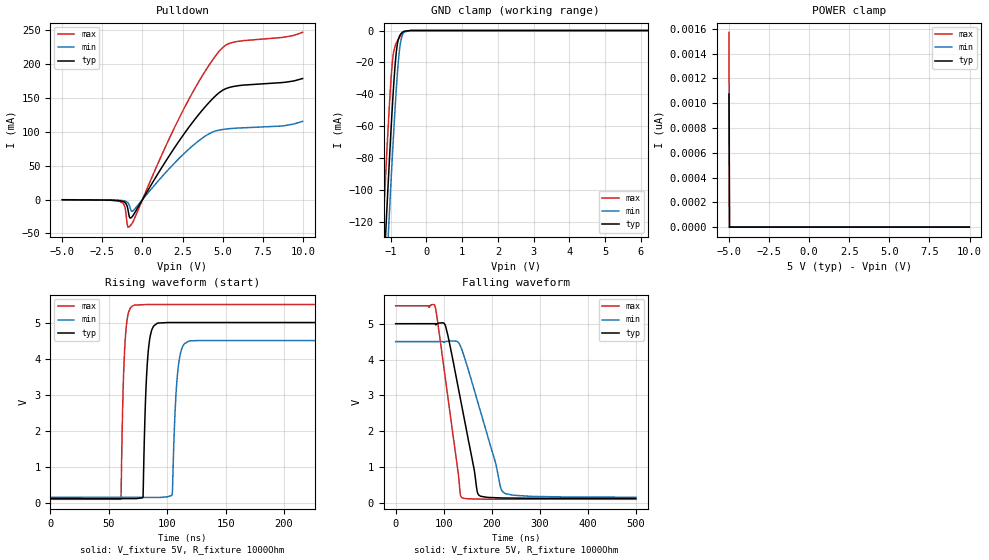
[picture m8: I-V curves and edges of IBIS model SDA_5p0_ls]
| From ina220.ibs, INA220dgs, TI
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|   Model
[Model]   SDA_5p0_ls
Model_type   I/O_open_drain
Polarity   Non-Inverting
Enable   Active-Low
Vinl = 1.5
Vinh = 3.5
Vmeas = 2.5
Vref = 5
Cref = 1pF
Rref = 1000
|   typ   min   max
C_comp   2.1193190E-12   1.8449300E-12 2.3639330E-12
[Voltage Range]   5   4.5   5.5
[Temperature Range]   27   85   -40
[Pullup Reference]   5   4.5   5.5
[Pulldown Reference]   -0   -0   -0
[Power Clamp Reference]   5   4.5   5.5
[GND Clamp Reference]   -0   -0   -0
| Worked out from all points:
|   slope of the pulldown table from 0 to 0.75 V, typ, clamps not added: 25.1 ohm
|   GND clamp passes 1 mA (typ) near -0.67 V on its own axis
|   falling waveform, V_fixture 5V, R_fixture 1000Ohm: 20-80 % time 42.4ns typ, 56.4ns min, 32.8ns max; typ from 5 V to 0.121 V
|   rising waveform, V_fixture 5V, R_fixture 1000Ohm: 20-80 % time 3.38ns typ, 3.94ns min, 2.89ns max; typ from 0.12 V to 5 V
[Pulldown]
|   Voltage   I(typ)   I(min)   I(max)
-5V       -196.2uA   -134.4uA   -251uA
-1.25V    -2.441mA   -1.382mA   -4.492mA
-1.085V   -4.401mA   -2.153mA   -12.11mA
-965mV    -9.014mA   -3.516mA   -34.28mA
-830mV    -24.29mA   -7.959mA   -40.07mA
-710mV    -26.92mA   -16.23mA   -37.21mA
-575mV    -23.01mA   -16.32mA   -31.97mA
2.47V     92.88mA    65.15mA    128.9mA
3.94V     137.8mA    94.18mA    190.8mA
4.78V     157.9mA    102.6mA    219mA
5.62V     166.8mA    105.1mA    232mA
9.985V    178.8mA    115.6mA    247mA
[GND Clamp]
|   Voltage   I(typ)   I(min)   I(max)
-5V       -2.019A    -2.05A     -1.986A
-1.25V    -176mA     -210.3mA   -138.9mA
-1.145V   -127.9mA   -162mA     -91.29mA
-1.1V     -107.8mA   -141.6mA   -71.72mA
-1.055V   -88.14mA   -121.6mA   -53.09mA
-965mV    -51.09mA   -82.91mA   -22.18mA
-920mV    -34.59mA   -64.52mA   -13.48mA
-860mV    -16.84mA   -41.85mA   -8.642mA
-800mV    -6.709mA   -22.67mA   -5.926mA
-740mV    -2.824mA   -9.434mA   -3.68mA
-620mV    -430.2uA   -885.3uA   -725.2uA
9.985V    0A         0A         0A
[POWER Clamp]
|   Voltage   I(typ)   I(min)   I(max)
-5V       1.074nA    0A         1.571nA
-4.97V    0A         0A         0A
-4.955V   0A         0A         0A
9.985V    0A         0A         0A
[Ramp]
R_load = 1000
|   typ   min   max
dV/dt_r   2.92774/3.37213e-09   2.60948/3.92775e-09   3.24271/2.87247e-09
dV/dt_f   2.9275/4.23604e-08   2.60776/5.64045e-08   3.24268/3.27444e-08
[Falling Waveform]
V_fixture = 5V
V_fixture_min = 4.5V
V_fixture_max = 5.5V
R_fixture = 1000Ohm
C_fixture = 0F
|   Time   V(typ)   V(min)   V(max)
0s        5V         4.5V       5.5V
80.83ns   5V         4.5V       5.528V
103.3ns   4.958V     4.498V     3.48V
134.4ns   2.93V      4.39V      252.5mV
137.9ns   2.684V     4.271V     142.4mV
171ns     255.5mV    2.804V     103.9mV
207.2ns   140.9mV    1.145V     100mV
219.5ns   134.4mV    378.7mV    99.82mV
224.6ns   132.1mV    286.4mV    99.75mV
500ns     120.8mV    153.7mV    95.53mV
[Rising Waveform]
V_fixture = 5V
V_fixture_min = 4.5V
V_fixture_max = 5.5V
R_fixture = 1000Ohm
C_fixture = 0F
|   Time   V(typ)   V(min)   V(max)
0s        120.4mV    150.9mV    95.49mV
60.41ns   116.6mV    149.2mV    96.06mV
64.16ns   116.3mV    149.1mV    4.543V
71.57ns   115.8mV    148.9mV    5.48V
79.36ns   170.6mV    148.7mV    5.495V
91.27ns   4.975V     148.4mV    5.5V
104.3ns   5V         238.3mV    5.5V
109.4ns   5V         3.735V     5.5V
118.6ns   5V         4.483V     5.5V
500ns     5V         4.5V       5.5V
